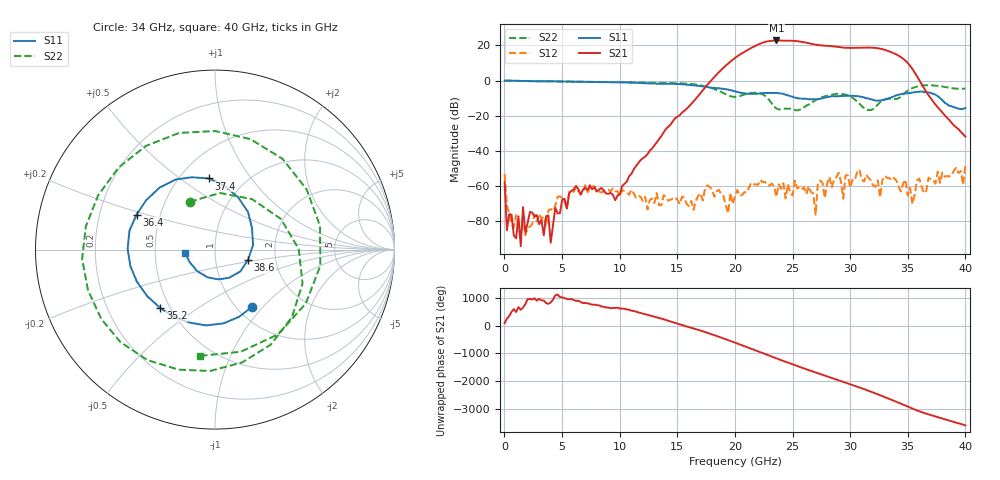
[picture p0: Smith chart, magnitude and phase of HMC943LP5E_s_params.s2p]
!Agilent Technologies,E8361A,US43140893,A.06.04.32
!Agilent HMC943LP5E: A.06.04.32
!Date: Wednesday, November 18, 2012 13:50:33
!Correction: S11(Full 2 Port(1,2)) S21(Full 2 Port(1,2)) S12(Full 2 Port(1,2)) S22(Full 2 Port(1,2))
!S2P File: Measurements: S11, S21, S12, S22:
# GHz S  dB  R 50
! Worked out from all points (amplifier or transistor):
!   201 points, 10 MHz to 40 GHz, reference 50 ohm
!   highest |S21| = 22.8 dB at 23.6 GHz (marker M1)
!   |S21| within 3 dB of that: 21.79 GHz to 27.77 GHz (5.984 GHz wide, 24.1 % of centre)
!   unconditionally stable (mu >= 1): start of sweep to end of sweep
!   at 6.61 GHz: K = 27986.25, MAG = -47.6 dB, |S12| = -64.5 dB
!   at 20.01 GHz: K = 144.15, MAG = 14.7 dB, |S12| = -65.6 dB
!   at 40 GHz: K = 3028.00, MAG = -29.8 dB, |S12| = -47.9 dB
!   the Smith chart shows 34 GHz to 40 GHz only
!   S11 on the Smith chart (normalised r, x): 34 GHz: 1.17, -0.87; 35.2 GHz: 0.44, -0.36; 36.4 GHz: 0.37, +0.19; 37.4 GHz: 0.69, +0.65; 38.6 GHz: 1.44, -0.17; 40 GHz: 0.71, -0.03
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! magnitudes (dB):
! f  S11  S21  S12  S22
! 10 MHz  0.0  -57.6  -53.1  -0.1
! 210 MHz  0.0  -85.0  -70.9  0.0
! 610 MHz  0.0  -76.1  -81.5  -0.1
! 4.21 GHz  -0.4  -82.3  -73.9  -0.4
! 6.81 GHz  -0.7  -61.9  -63.5  -0.7
! 9.61 GHz  -0.9  -67.9  -62.8  -0.8
! 13.41 GHz  -1.8  -33.4  -70.8  -1.2
! 20.01 GHz  -6.1  12.9  -65.6  -9.3
! 23.6 GHz  -7.0  22.8  -66.0  -15.8
! 26.8 GHz  -10.7  20.6  -64.0  -11.9
! 27 GHz  -10.7  20.4  -76.1  -11.1
! 27.4 GHz  -10.3  20.0  -56.7  -9.7
! 29 GHz  -8.8  19.1  -52.4  -7.6
! 29.4 GHz  -8.7  18.8  -67.0  -7.7
! 29.6 GHz  -8.6  18.6  -53.8  -7.9
! 33.4 GHz  -10.0  16.6  -55.4  -10.3
! 34 GHz  -8.4  14.9  -56.7  -10.4
! 35.2 GHz  -7.0  8.4  -61.0  -4.9
! 36.4 GHz  -6.4  -4.1  -63.9  -2.6
! 37.4 GHz  -8.0  -13.6  -58.5  -2.9
! 38.6 GHz  -14.3  -22.3  -54.4  -4.0
! 40 GHz  -15.6  -31.8  -47.9  -4.5
